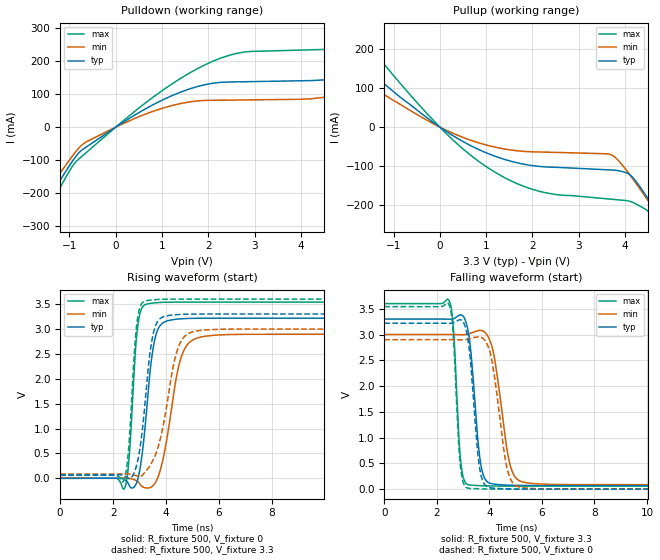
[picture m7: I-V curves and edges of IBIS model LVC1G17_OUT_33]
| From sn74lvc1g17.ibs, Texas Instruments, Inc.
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[Model]   LVC1G17_OUT_33
Model_type  Output
Vref =   0
Rref =   500
Cref =   50p
Vmeas =   1.5
| variable   typ   min   max
C_comp   9.41pF   5.86pF   12.60pF
| C_pullup   9.85pF   5.86pF   11.96pF
| C_pulldown   8.97pF   6.16pF   12.60pF
[Temperature Range]   40   100   -40
| Ambient temperature   25   85   -40
[Voltage range]   3.3   3   3.6
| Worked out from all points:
|   slope of the pulldown table from 0 to 0.495 V, typ, clamps not added: 11.3 ohm
|   slope of the pullup table from 0 to 0.495 V, typ, clamps not added: 13.6 ohm
|   rising waveform, R_fixture 500, V_fixture 0: 20-80 % time 368ps typ, 551ps min, 241ps max; typ from 0 V to 3.22 V
|   falling waveform, R_fixture 500, V_fixture 3.3: 20-80 % time 314ps typ, 471ps min, 210ps max; typ from 3.3 V to 0.069 V
|   rising waveform, R_fixture 500, V_fixture 3.3: 20-80 % time 385ps typ, 622ps min, 245ps max; typ from 0.069 V to 3.3 V
|   falling waveform, R_fixture 500, V_fixture 0: 20-80 % time 305ps typ, 452ps min, 208ps max; typ from 3.22 V to 0 V
[Pulldown]
| LVC1G17_OUT_33
|   Voltage   I(typ)   I(min)   I(max)
-5.5V     -1.112A    -993.8mA   -1.259A
-2.645V   -490.3mA   -433.2mA   -553.8mA
-1.49V    -226.9mA   -197.7mA   -257.3mA
-540mV    -51.04mA   -37.69mA   -65.27mA
1.025V    83.38mA    58mA       112.9mA
2.285V    136mA      81.66mA    210.1mA
4.75V     148.7mA    96.8mA     237.9mA
6.98V     278.7mA    201.6mA    396.3mA
7.35V     308.5mA    129.4mA    437mA
7.84V     330.1mA    92.52mA    494.2mA
8.75V     170.8mA    93.27mA    500.6mA
11V       160mA      96.49mA    276.8mA
[Pullup]
| LVC1G17_OUT_33
|   Voltage   I(typ)   I(min)   I(max)
-5.5V     609.5mA    479.2mA    854.2mA
-3.13V    322.5mA    249.3mA    458mA
-2.385V   237.2mA    181.8mA    339.2mA
-1.845V   177.9mA    135.2mA    255.8mA
-130mV    10.97mA    8.025mA    16.16mA
1.04V     -67.46mA   -46.7mA    -103.9mA
2.145V    -100.4mA   -63.42mA   -163.8mA
3.71V     -109.5mA   -71.26mA   -184.2mA
4.15V     -126.7mA   -129.5mA   -191.6mA
4.765V    -233mA     -235.6mA   -263.4mA
4.95V     -268.4mA   -268.9mA   -301.3mA
11V       -1.523A    -1.428A    -1.684A
[Ramp]
| LVC1G17_OUT_33
| variable   typ   min   max
dV/dt_r   2.05/3.96E-10   1.85/5.96E-10   2.25/2.66E-10
dV/dt_f   1.99/3.33E-10   1.80/4.93E-10   2.18/2.25E-10
R_load = 500
[Rising Waveform]
| LVC1G17_OUT_33
R_fixture =   500
C_fixture =   0
L_fixture =   0
V_fixture =   0
V_fixture_min = 0
V_fixture_max = 0
|   Time   V(typ)   V(min)   V(max)
0s        141.7pV    4.978nV    2.659nV
2.435ns   -31.15mV   4.425mV    -199.5mV
2.6ns     -130.3mV   1.091mV    384.7mV
2.92ns    -39.9mV    -61.43mV   3.009V
3.285ns   1.486V     -195.4mV   3.501V
3.495ns   2.558V     -153.5mV   3.519V
3.735ns   3.036V     83.64mV    3.531V
4.535ns   3.203V     2.367V     3.538V
5.22ns    3.214V     2.825V     3.539V
23.6ns    3.216V     2.894V     3.539V
[Falling Waveform]
| LVC1G17_OUT_33
R_fixture =   500
C_fixture =   0
L_fixture =   0
V_fixture =   3.3
V_fixture_min = 3
V_fixture_max = 3.6
|   Time   V(typ)   V(min)   V(max)
0s        3.3V       3V         3.6V
2.48ns    3.296V     3V         3.642V
2.64ns    3.308V     3V         3.052V
2.905ns   3.381V     2.996V     560.8mV
3.205ns   3.028V     3.011V     83.8mV
3.65ns    560.7mV    3.081V     67.84mV
4.025ns   114.6mV    2.88V      62.07mV
4.765ns   76.93mV    521.3mV    59.49mV
5.28ns    71.86mV    136.9mV    59.16mV
23.6ns    69.39mV    85.93mV    58.96mV
[Rising Waveform]
| LVC1G17_OUT_33
R_fixture =   500
C_fixture =   0
L_fixture =   0
V_fixture =   3.3
V_fixture_min = 3
V_fixture_max = 3.6
|   Time   V(typ)   V(min)   V(max)
0s        69.35mV    85.87mV    58.92mV
2.4ns     51.78mV    89.64mV    -47.43mV
2.58ns    -5.569mV   88.16mV    557.9mV
2.895ns   275.8mV    49.41mV    3.095V
3.21ns    1.533V     124.9mV    3.564V
3.42ns    2.623V     277.8mV    3.58V
3.665ns   3.137V     570mV      3.591V
4.405ns   3.287V     2.539V     3.599V
5.015ns   3.298V     2.943V     3.6V
23.6ns    3.3V       3V         3.6V
[Falling Waveform]
| LVC1G17_OUT_33
R_fixture =   500
C_fixture =   0
L_fixture =   0
V_fixture =   0
V_fixture_min = 0
V_fixture_max = 0
|   Time   V(typ)   V(min)   V(max)
0s        3.22V      2.9V       3.542V
2.465ns   3.217V     2.9V       3.576V
2.615ns   3.225V     2.9V       3.07V
2.895ns   3.286V     2.897V     456.2mV
3.19ns    2.888V     2.91V      17.92mV
3.61ns    476.7mV    2.954V     7.832mV
3.995ns   32.14mV    2.707V     2.716mV
4.66ns    6.332mV    435.2mV    587.8uV
5.125ns   2.227mV    43.64mV    260.3uV
23.6ns    38.64uV    48.8uV     36.05uV
